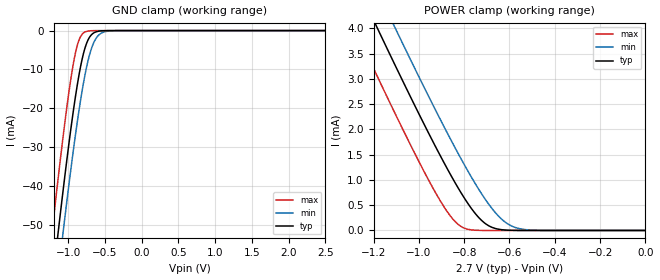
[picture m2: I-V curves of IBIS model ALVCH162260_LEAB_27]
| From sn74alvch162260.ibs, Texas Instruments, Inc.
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[Model]   ALVCH162260_LEAB_27
Model_type  Input
Vinl=0.8
Vinh=2.0
| variable   typ   min   max
C_comp   1.72pF   1.58pF   1.83pF
[Temperature Range]   40   100   -40
| Ambient temperature   25   85   -40
[Voltage range]   2.7   2.7   2.7
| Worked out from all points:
|   GND clamp passes 1 mA (typ) near -0.68 V on its own axis
|   POWER clamp passes 1 mA (typ) near -0.85 V on its own axis
[GND Clamp]
| ALVCH162260_LEAB_27
|   Voltage   I(typ)   I(min)   I(max)
-2.5V     -300mA     -309.4mA   -288.3mA
-1.22V    -65.92mA   -76.78mA   -51.96mA
-1.15V    -54.2mA    -65.07mA   -40.19mA
-1.125V   -50.1mA    -60.96mA   -36.1mA
-1.07V    -41.27mA   -52.08mA   -27.39mA
-980mV    -27.63mA   -38.14mA   -14.46mA
-910mV    -18.08mA   -28.05mA   -6.523mA
-845mV    -10.58mA   -19.54mA   -2.069mA
-780mV    -5.041mA   -12.24mA   -440.8uA
-655mV    -630uA     -3.209mA   -15.41uA
-485mV    -21.18uA   -229.3uA   -148.8nA
2.5V      1.112nA    1.808uA    4.19pA
[POWER Clamp]
| ALVCH162260_LEAB_27
|   Voltage   I(typ)   I(min)   I(max)
-2.7V     18.86mA    19.56mA    17.97mA
-1.3V     5.111mA    5.849mA    4.158mA
-1.255V   4.681mA    5.42mA     3.727mA
-1.17V    3.877mA    4.616mA    2.921mA
-1.1V     3.223mA    3.962mA    2.267mA
-935mV    1.732mA    2.457mA    816uA
-840mV    943.8uA    1.634mA    176.2uA
-795mV    611.2uA    1.266mA    38.41uA
-725mV    207uA      738.7uA    1.527uA
-625mV    11.21uA    186.8uA    11.91nA
-510mV    181.6nA    9.688uA    51.12pA
-35.59fV  5.11pA     7.205pA    4.886pA
